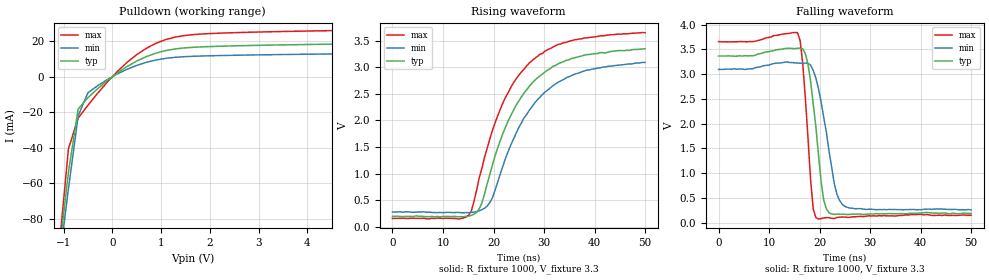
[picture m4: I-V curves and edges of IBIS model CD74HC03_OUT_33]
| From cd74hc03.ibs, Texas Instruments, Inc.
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|   Model CD74HC03 OUTPUT_33
[Model]   CD74HC03_OUT_33
Model_type  Open_drain
Polarity   Non-Inverting
Vref = 3.3
Rref = 1000
Cref = 50p
Vmeas = 1.65
| variable   typ   min   max
C_comp   1.930pf   1.534pf   2.323pf
[Temperature Range]   25   85   -40
[Voltage range]   3.3   3.0   3.6
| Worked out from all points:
|   slope of the pulldown table from 0 to 0.495 V, typ, clamps not added: 56.5 ohm
|   rising waveform, R_fixture 1000, V_fixture 3.3: 20-80 % time 9ns typ, 9.3ns min, 8.89ns max; typ from 0.196 V to 3.35 V
|   falling waveform, R_fixture 1000, V_fixture 3.3: 20-80 % time 1.94ns typ, 2.73ns min, 1.37ns max; typ from 3.37 V to 0.187 V
[Pulldown]
|   Voltage   I(typ)   I(min)   I(max)
-3.3V     -624mA     -584mA     -740.9mA
-1.1V     -101.4mA   -106.6mA   -98.93mA
-900mV    -53.85mA   -63.21mA   -40.57mA
-700mV    -18.17mA   -22.03mA   -23.31mA
-500mV    -11.83mA   -9.02mA    -16.09mA
-100mV    -2.127mA   -1.572mA   -2.957mA
300mV     5.686mA    4.129mA    7.989mA
500mV     8.798mA    6.336mA    12.42mA
900mV     13.3mA     9.428mA    18.88mA
1.3V      15.68mA    10.94mA    22.36mA
1.9V      16.87mA    11.7mA     24.14mA
6.6V      19.14mA    13.48mA    26.88mA
[ramp]
| variable   typ   min   max
dV/dt_r   1.932E+00/8.575E-09  1.722E+00/8.927E-09  2.144E+00/8.386E-09
dV/dt_f   1.956E+00/1.845E-09  1.746E+00/2.634E-09  2.160E+00/1.296E-09
[Rising Waveform]
R_fixture = 1000
V_fixture = 3.3
V_fixture_min = 3.0
V_fixture_max = 3.6
C_fixture = 0
L_fixture = 0
|   Time   V(typ)   V(min)   V(max)
0s        196.2mV    275.7mV    156.6mV
15.1ns    199.3mV    262.6mV    218.5mV
15.63ns   214.8mV    269.5mV    302.6mV
17.19ns   343.2mV    300mV      926.4mV
19.27ns   983.4mV    454.9mV    1.654V
21.88ns   1.759V     1.149V     2.335V
26.04ns   2.515V     2.049V     2.963V
29.17ns   2.838V     2.435V     3.245V
35.94ns   3.176V     2.867V     3.514V
50ns      3.349V     3.091V     3.65V
[Falling Waveform]
R_fixture = 1000
V_fixture = 3.3
V_fixture_min = 3.0
V_fixture_max = 3.6
C_fixture = 0
L_fixture = 0
|   Time   V(typ)   V(min)   V(max)
0s        3.368V     3.097V     3.66V
15.63ns   3.525V     3.226V     3.841V
16.67ns   3.514V     3.223V     3.22V
17.71ns   3.201V     3.221V     1.716V
18.75ns   2.399V     3.078V     277.9mV
19.27ns   1.942V     2.922V     104.5mV
20.83ns   455.3mV    2.126V     96.28mV
22.92ns   166.9mV    787.8mV    84.38mV
24.48ns   170.9mV    370.5mV    113.8mV
50ns      187.1mV    257mV      151.2mV
